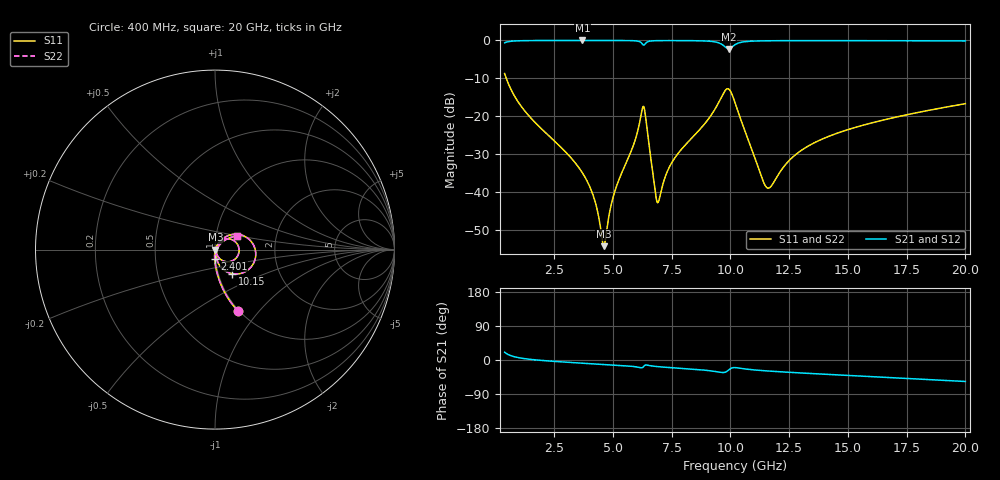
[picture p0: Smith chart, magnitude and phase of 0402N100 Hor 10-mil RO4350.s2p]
# GHz S MA R 50
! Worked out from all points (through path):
!   1960 points, 400 MHz to 20 GHz, reference 50 ohm
!   highest |S21| = -0.02 dB at 3.712 GHz (marker M1); lowest = -2.2 dB at 9.925 GHz (marker M2)
!   group delay of S21, straight-line fit = 8.45 ps
!   lowest |S11| = -54.4 dB at 4.622 GHz (marker M3), VSWR 1.00, Z = 50.2 - j0.0419 ohm
!   |S11| at or under -10 dB: 469.3 MHz to end of sweep
!   |S22| runs from -54.4 to -8.8 dB; largest |S21 - S12| = 0
!   S11 on the Smith chart (normalised r, x): 400 MHz: 0.99, -0.78; 2.401 GHz: 0.99, -0.10; 10.15 GHz: 1.17, -0.32; 20 GHz: 1.27, +0.20
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0.4  0.3649 -69.5  0.9306 20.4  0.9306 20.4  0.3649 -69.5
1.130373  0.1316 -85.0  0.9905 4.7  0.9905 4.7  0.1316 -85.0
2.401021  0.05073 -91.9  0.9975 -3.2  0.9975 -3.2  0.05073 -91.9
3.671669  0.01853 -93.6  0.9982 -8.2  0.9982 -8.2  0.01853 -93.6
3.71169  0.01773 -93.5  0.9982 -8.4  0.9982 -8.4  0.01773 -93.5
4.211945  0.008116 -88.1  0.9981 -10.2  0.9981 -10.2  0.008116 -88.1
4.622154  0.001913 -12.6  0.9979 -11.7  0.9979 -11.7  0.001913 -12.6
5.062379  0.009535 62.5  0.9974 -13.3  0.9974 -13.3  0.009535 62.5
5.902808  0.04323 61.2  0.9902 -17.3  0.9902 -17.3  0.04323 61.2
6.283002  0.1322 6.7  0.8791 -19.2  0.8791 -19.2  0.1322 6.7
6.403063  0.09437 -46.1  0.9192 -13.2  0.9192 -13.2  0.09437 -46.1
6.813272  0.009593 -43.4  0.9911 -16.9  0.9911 -16.9  0.009593 -43.4
6.943338  0.007377 8.0  0.9931 -17.7  0.9931 -17.7  0.007377 8.0
7.57366  0.02612 59.2  0.9947 -20.5  0.9947 -20.5  0.02612 59.2
9.51465  0.1531 33.9  0.9269 -31.9  0.9269 -31.9  0.1531 33.9
9.92486  0.2283 -18.8  0.7729 -26.6  0.7729 -26.6  0.2283 -18.8
10.15498  0.1654 -54.4  0.8586 -20.0  0.8586 -20.0  0.1654 -54.4
10.205  0.1491 -59.5  0.8799 -20.1  0.8799 -20.1  0.1491 -59.5
11.5757  0.01124 -22.2  0.9884 -28.9  0.9884 -28.9  0.01124 -22.2
13.46667  0.04271 46.6  0.9929 -35.8  0.9929 -35.8  0.04271 46.6
16.73834  0.0922 40.9  0.9905 -46.3  0.9905 -46.3  0.0922 40.9
20  0.1459 31.5  0.9838 -56.7  0.9838 -56.7  0.1459 31.5
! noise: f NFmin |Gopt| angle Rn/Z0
0.4  0.001103  0.7594  1.874  0.0009287
2.571  0.004612  0.6523  6.756  0.002515
4.752  0.008098  0.6385  12  0.004182
6.933  0.01768  0.7446  17.46  0.01359
9.104  0.03475  0.8234  22.73  0.03971
11.29  0.0324  0.7741  28.15  0.02759
13.47  0.02247  0.6446  33.11  0.01105
15.64  0.02216  0.5993  37.85  0.009177
17.82  0.02328  0.5786  42.46  0.008818
20  0.02488  0.5685  46.9  0.008886
